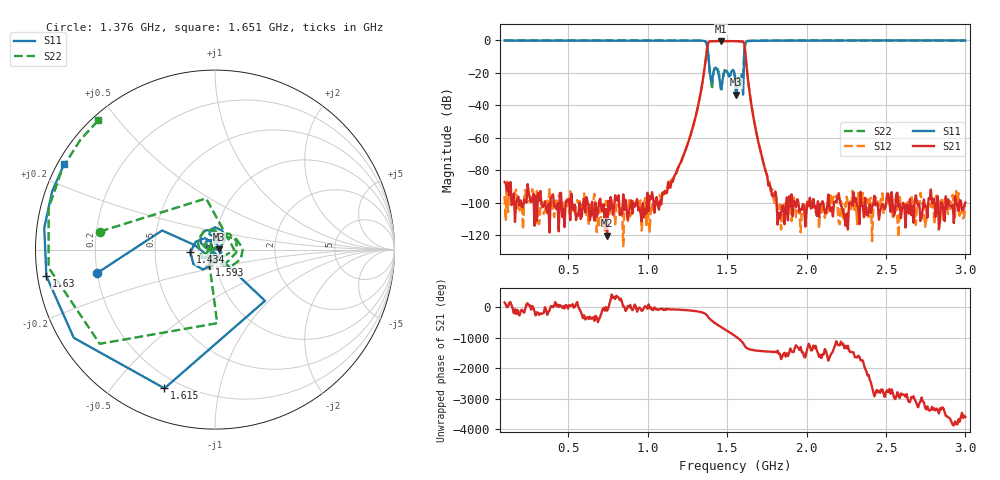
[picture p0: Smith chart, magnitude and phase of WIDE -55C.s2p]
!Agilent Technologies,E8364B,MY43040699,A.07.50.67
!Agilent E8364B: A.07.50.67
!Date: Wednesday, June 25, 2025 05:53:14
!Correction: S11(Full 2 Port(1,2))
!S21(Full 2 Port(1,2))
!S12(Full 2 Port(1,2))
!S22(Full 2 Port(1,2))
!S2P File: Measurements: S11, S21, S12, S22:
# Hz S  dB  R 50
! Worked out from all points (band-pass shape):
!   401 points, 100 MHz to 3 GHz, reference 50 ohm
!   highest |S21| = -0.40 dB at 1.463 GHz (marker M1); lowest = -120.2 dB at 745.2 MHz (marker M2)
!   |S21| within 3 dB of the highest: 1.377 GHz to 1.61 GHz (232.3 MHz wide, 15.6 % of centre)
!   lowest |S11| = -33.4 dB at 1.557 GHz (marker M3), VSWR 1.04, Z = 52.2 + j0.27 ohm
!   |S11| at or under -10 dB: 1.383 GHz to 1.607 GHz (224.3 MHz wide, 15 % of centre)
!   |S22| runs from -34.2 to 0.0 dB; largest |S21 - S12| = 0.00091
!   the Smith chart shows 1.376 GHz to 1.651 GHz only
!   S11 on the Smith chart (normalised r, x): 1.376 GHz: 0.20, -0.09; 1.434 GHz: 0.76, -0.02; 1.593 GHz: 0.93, -0.16; 1.615 GHz: 0.14, -0.69; 1.63 GHz: 0.03, -0.08; 1.651 GHz: 0.02, +0.26
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1e8  -0.07 168.7  -87.26 166.6  -95.88 146.1  -0.04 168.6
5.8575e8  -0.13 112.2  -108.38 132.7  -100.76 11.0  -0.11 112.2
7.4525e8  -0.12 92.9  -120.21 -104.4  -98.94 -73.9  -0.10 93.1
1.0715e9  -0.08 45.1  -104.25 -63.9  -95.08 -50.4  -0.08 47.6
1.22375e9  -0.06 7.3  -71.42 -80.3  -71.16 -81.2  -0.07 13.0
1.347e9  -0.21 -79.5  -24.84 -168.5  -24.84 -168.5  -0.21 -71.8
1.376e9  -3.48 -168.7  -3.92 86.1  -3.92 86.1  -3.76 171.1
1.41225e9  -20.74 -104.3  -0.49 -108.4  -0.49 -108.4  -21.55 62.5
1.434e9  -17.22 -174.5  -0.51 171.8  -0.51 171.8  -16.28 -19.8
1.463e9  -30.14 144.8  -0.40 74.7  -0.40 74.7  -31.60 -168.4
1.48475e9  -19.09 135.7  -0.45 4.6  -0.45 4.6  -18.45 47.6
1.51375e9  -22.10 100.3  -0.43 -88.8  -0.43 -88.8  -22.23 -97.5
1.55e9  -22.30 43.7  -0.47 146.6  -0.47 146.6  -22.57 65.0
1.55725e9  -33.43 7.0  -0.47 119.3  -0.46 119.4  -34.20 47.6
1.5935e9  -21.03 -110.5  -0.68 -43.1  -0.68 -43.1  -20.88 -150.3
1.61525e9  -1.70 -110.0  -7.91 150.0  -7.91 150.0  -1.62 -140.7
1.62975e9  -0.44 -171.1  -22.44 91.1  -22.43 91.1  -0.40 166.0
1.6515e9  -0.29 150.5  -38.72 54.1  -38.71 54.1  -0.26 132.1
1.74575e9  -0.16 90.6  -81.53 1.0  -81.49 -3.8  -0.14 78.2
2.03575e9  -0.08 32.9  -102.68 33.8  -96.99 50.5  -0.07 24.7
2.5215e9  -0.05 -15.6  -98.87 -156.4  -101.01 141.2  -0.05 -22.3
3e9  -0.04 -52.6  -99.79 6.6  -101.66 169.0  -0.04 -58.6
